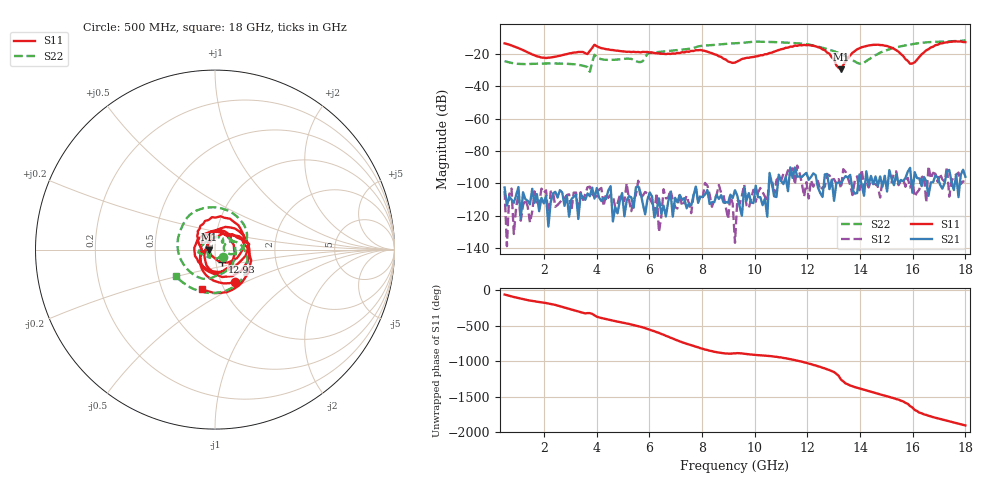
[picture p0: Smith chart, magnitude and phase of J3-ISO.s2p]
!Agilent Technologies,N5230C,MY49001096,A.09.42.15
!Agilent N5230C: A.09.42.15
!Date: Thursday, June 29, 2023 08:12:34
!Correction: S11(Full 2 Port(1,2))
!S21(Full 2 Port(1,2))
!S12(Full 2 Port(1,2))
!S22(Full 2 Port(1,2))
!S2P File: Measurements: S11, S21, S12, S22:
# Hz S  dB  R 50
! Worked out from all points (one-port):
!   201 points, 500 MHz to 18 GHz, reference 50 ohm
!   lowest |S11| = -29.4 dB at 13.28 GHz (marker M1), VSWR 1.07, Z = 46.7 - j0.0164 ohm
!   |S11| at or under -10 dB: start of sweep to end of sweep
!   S11 on the Smith chart (normalised r, x): 500 MHz: 1.17, -0.44; 12.93 GHz: 1.07, -0.15; 18 GHz: 0.79, -0.37
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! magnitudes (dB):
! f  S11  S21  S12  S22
! 500 MHz  -13.4  -102.6  -104.8  -24.4
! 1.9 GHz  -22.2  -109.0  -103.2  -26.0
! 3.475 GHz  -18.8  -108.7  -110.3  -27.3
! 3.65 GHz  -20.0  -106.2  -102.4  -28.1
! 3.737 GHz  -18.0  -108.0  -102.1  -31.0
! 3.913 GHz  -14.3  -109.4  -108.2  -20.5
! 4.263 GHz  -16.7  -108.9  -114.2  -23.5
! 5.662 GHz  -19.0  -105.8  -109.1  -25.0
! 5.925 GHz  -18.7  -110.0  -106.3  -20.0
! 6.362 GHz  -19.7  -109.3  -130.1  -18.7
! 7.938 GHz  -17.6  -108.3  -107.1  -15.1
! 9.25 GHz  -25.3  -104.3  -136.8  -13.3
! 11.53 GHz  -14.8  -90.2  -100.8  -13.3
! 12.22 GHz  -15.0  -93.9  -102.1  -14.8
! 12.93 GHz  -22.1  -97.7  -98.0  -17.8
! 13.28 GHz  -29.4  -100.2  -103.1  -20.0
! 13.54 GHz  -22.4  -96.4  -96.6  -22.1
! 13.97 GHz  -16.5  -94.5  -104.3  -26.0
! 15.11 GHz  -15.6  -91.8  -98.7  -17.0
! 15.9 GHz  -26.0  -90.4  -102.6  -14.2
! 16.86 GHz  -14.5  -95.0  -94.1  -12.5
! 18 GHz  -12.6  -95.9  -99.2  -11.6
